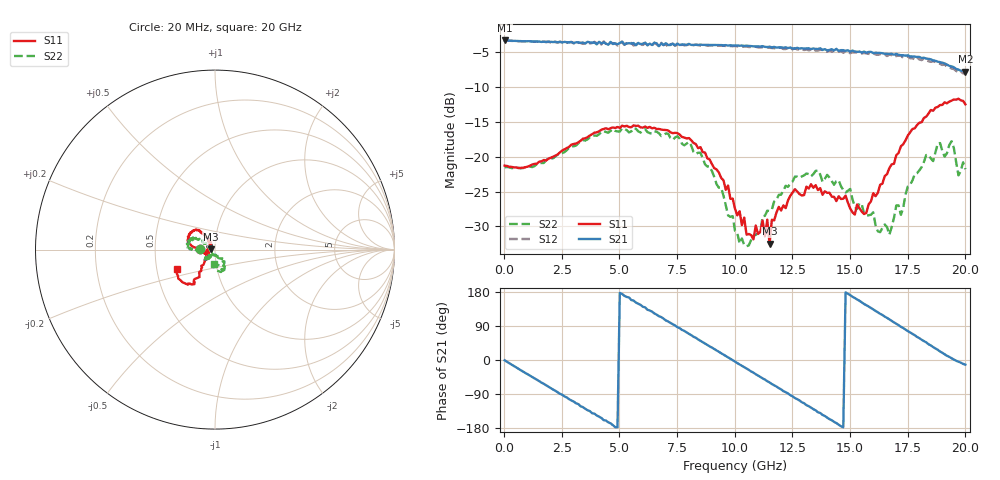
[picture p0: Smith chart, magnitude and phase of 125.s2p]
!Agilent Technologies,N5230A,US43500223,A.07.50.48
!Agilent N5230A: A.07.50.48
!Date: Wednesday, October 07, 2015 19:48:35
!Correction: S11(Full 2 Port(1,2))
!S21(Full 2 Port(1,2))
!S12(Full 2 Port(1,2))
!S22(Full 2 Port(1,2))
!S2P File: Measurements: S11, S21, S12, S22:
# Hz S  RI  R 50
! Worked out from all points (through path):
!   201 points, 20 MHz to 20 GHz, reference 50 ohm
!   highest |S21| = -3.32 dB at 20 MHz (marker M1); lowest = -7.8 dB at 20 GHz (marker M2)
!   group delay of S21, straight-line fit = 102 ps
!   lowest |S11| = -32.5 dB at 11.51 GHz (marker M3), VSWR 1.05, Z = 47.7 + j0.063 ohm
!   |S11| at or under -10 dB: start of sweep to end of sweep
!   |S22| runs from -32.8 to -15.9 dB; largest |S21 - S12| = 0.032
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2e7  -0.0863 0.0013  0.6825 -0.00944  0.6807 -0.0101  -0.0839 0.000874
1.9181e9  -0.0967 0.00536  0.2217 -0.6322  0.2156 -0.6313  -0.0972 -0.000816
3.4166e9  -0.1328 0.0233  -0.3722 -0.5447  -0.3644 -0.5323  -0.1315 -0.00105
5.1149e9  -0.1511 0.0713  -0.6675 0.0678  -0.6603 0.0736  -0.1564 0.033
6.7133e9  -0.1156 0.1081  -0.2678 0.5599  -0.2653 0.5602  -0.1385 0.0498
8.012e9  -0.0853 0.1061  0.2321 0.6022  0.2382 0.5914  -0.1103 0.0644
9.4106e9  -0.0344 0.0615  0.6015 0.1948  0.5988 0.1844  -0.0518 0.0301
1.001e10  -0.0274 0.0322  0.6265 -0.0451  0.6207 -0.053  -0.0293 0.0022
1.06094e10  -0.0197 0.0198  0.5603 -0.2745  0.543 -0.2828  -0.0189 -0.0133
1.13087e10  -0.0259 0.00722  0.3809 -0.4813  0.3638 -0.4801  -0.0196 -0.0323
1.14086e10  -0.0349 0.00551  0.3425 -0.5075  0.334 -0.511  -0.0206 -0.0355
1.15085e10  -0.0237 0.00066  0.3161 -0.5284  0.298 -0.526  -0.0241 -0.0329
1.19081e10  -0.0434 -0.00466  0.1659 -0.5862  0.1523 -0.5873  -0.0286 -0.0449
1.34066e10  -0.0569 -0.0189  -0.3823 -0.4598  -0.3827 -0.452  -0.0536 -0.0525
1.49051e10  -0.0444 -0.0148  -0.5776 0.0526  -0.5608 0.0646  -0.0446 -0.0355
1.57043e10  -0.0357 -0.0169  -0.4557 0.3234  -0.4371 0.3359  -0.0249 -0.0283
1.67033e10  -0.0574 -0.0598  -0.1609 0.5219  -0.1528 0.5184  0.000398 -0.0276
1.75025e10  -0.0768 -0.1192  0.1267 0.5189  0.1263 0.5105  0.0352 -0.0501
1.88012e10  -0.122 -0.1923  0.4285 0.2184  0.4229 0.1932  0.0516 -0.1135
1.94006e10  -0.1717 -0.1857  0.4435 0.0353  0.429 0.0213  0.0333 -0.1248
1.97003e10  -0.2048 -0.1612  0.42 -0.032  0.4011 -0.0515  0.00175 -0.0735
2e10  -0.2109 -0.1097  0.3975 -0.0865  0.3818 -0.1044  -0.00463 -0.0812
